FUNCTION "OutputsLoader" : VOID
TITLE =Outputs loader
//Network 1-3 is the startup sequence for the robot cabinet and must not be
//changed in any way
VERSION : 0.1

BEGIN
NETWORK
TITLE =Reset emergency stop loaderside
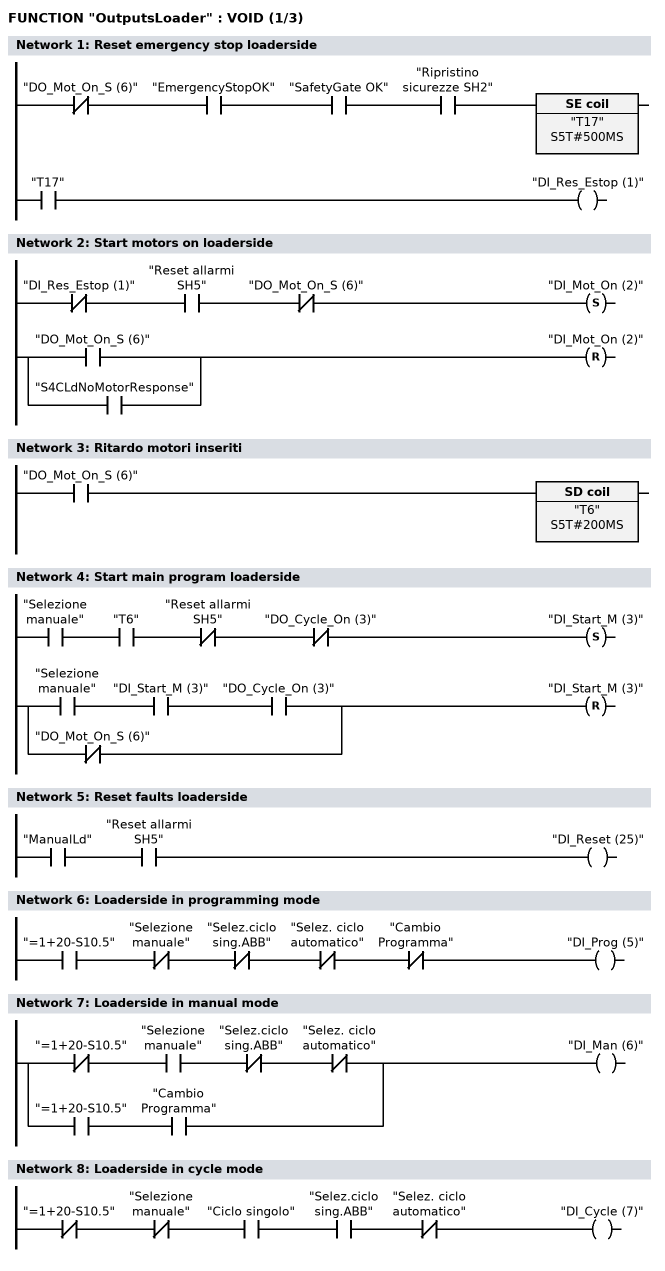
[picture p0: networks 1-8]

      UN    "DO_Mot_On_S (6)";
      U     "EmergencyStopOK";
      U     "SafetyGate OK";
      U     "Ripristino sicurezze SH2";
      L     S5T#500MS;
      SV    "T17";
      NOP   0;
      NOP   0;
      NOP   0;
      U     "T17";
      =     "DI_Res_Estop (1)";
NETWORK
TITLE =Start motors on loaderside

      UN    "DI_Res_Estop (1)";
      U     "Reset allarmi SH5";
      UN    "DO_Mot_On_S (6)";
      S     "DI_Mot_On (2)";
      U(    ;
      O     "DO_Mot_On_S (6)";
      O     "S4CLdNoMotorResponse";
      )     ;
      R     "DI_Mot_On (2)";
      NOP   0;
NETWORK
TITLE =Ritardo motori inseriti

      U     "DO_Mot_On_S (6)";
      L     S5T#200MS;
      SE    "T6";
NETWORK
TITLE =Start main program loaderside

      U     "Selezione manuale";
      U     "T6";
      UN    "Reset allarmi SH5";
      UN    "DO_Cycle_On (3)";
      S     "DI_Start_M (3)";
      U(    ;
      U     "Selezione manuale";
      U     "DI_Start_M (3)";
      U     "DO_Cycle_On (3)";
      ON    "DO_Mot_On_S (6)";
      )     ;
      R     "DI_Start_M (3)";
      NOP   0;
NETWORK
TITLE =Reset faults loaderside

      U     "ManualLd";
      U     "Reset allarmi SH5";
      =     "DI_Reset (25)";
NETWORK
TITLE =Loaderside in programming mode

      U     "=1+20-S10.5";
      UN    "Selezione manuale";
      UN    "Selez.ciclo sing.ABB";
      UN    "Selez. ciclo automatico";
      UN    "Cambio Programma";
      =     "DI_Prog (5)";
NETWORK
TITLE =Loaderside in manual mode

      UN    "=1+20-S10.5";
      U     "Selezione manuale";
      UN    "Selez.ciclo sing.ABB";
      UN    "Selez. ciclo automatico";
      O     ;
      U     "=1+20-S10.5";
      U     "Cambio Programma";
      =     "DI_Man (6)";
NETWORK
TITLE =Loaderside in cycle mode

      UN    "=1+20-S10.5";
      UN    "Selezione manuale";
      U     "Ciclo singolo";
      U     "Selez.ciclo sing.ABB";
      UN    "Selez. ciclo automatico";
      =     "DI_Cycle (7)";
NETWORK
TITLE =Loaderside in auto mode
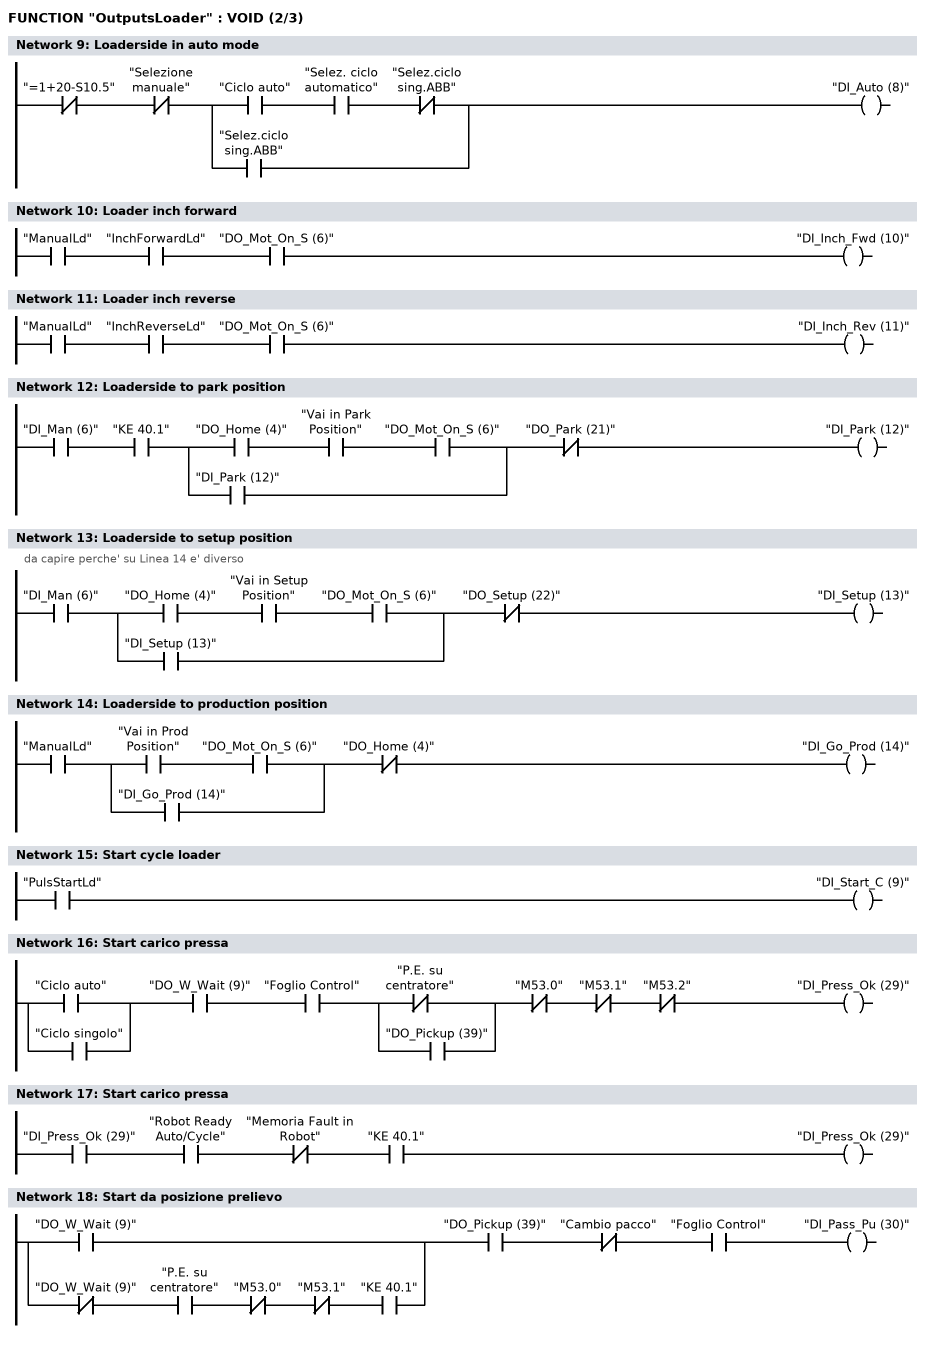
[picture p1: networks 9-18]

      UN    "=1+20-S10.5";
      UN    "Selezione manuale";
      U(    ;
      U     "Ciclo auto";
      U     "Selez. ciclo automatico";
      UN    "Selez.ciclo sing.ABB";
      O     "Selez.ciclo sing.ABB";
      )     ;
      =     "DI_Auto (8)";
NETWORK
TITLE =Loader inch forward

      U     "ManualLd";
      U     "InchForwardLd";
      U     "DO_Mot_On_S (6)";
      =     "DI_Inch_Fwd (10)";
NETWORK
TITLE =Loader inch reverse

      U     "ManualLd";
      U     "InchReverseLd";
      U     "DO_Mot_On_S (6)";
      =     "DI_Inch_Rev (11)";
NETWORK
TITLE =Loaderside to park position

      U     "DI_Man (6)";
      U     "KE 40.1";
      U(    ;
      U     "DO_Home (4)";
      U     "Vai in Park Position";
      U     "DO_Mot_On_S (6)";
      O     "DI_Park (12)";
      )     ;
      UN    "DO_Park (21)";
      =     "DI_Park (12)";
NETWORK
TITLE =Loaderside to setup position
//da capire perche' su Linea 14 e' diverso
      U     "DI_Man (6)";
      U(    ;
      U     "DO_Home (4)";
      U     "Vai in Setup Position";
      U     "DO_Mot_On_S (6)";
      O     "DI_Setup (13)";
      )     ;
      UN    "DO_Setup (22)";
      =     "DI_Setup (13)";
NETWORK
TITLE =Loaderside to production position

      U     "ManualLd";
      U(    ;
      U     "Vai in Prod Position";
      U     "DO_Mot_On_S (6)";
      O     "DI_Go_Prod (14)";
      )     ;
      UN    "DO_Home (4)";
      =     "DI_Go_Prod (14)";
NETWORK
TITLE =Start cycle loader

      U     "PulsStartLd";
      =     "DI_Start_C (9)";
NETWORK
TITLE =Start carico pressa

      U(    ;
      O     "Ciclo auto";
      O     "Ciclo singolo";
      )     ;
      U     "DO_W_Wait (9)";
      U     "Foglio Control";
      U(    ;
      ON    "P.E. su centratore";
      O     "DO_Pickup (39)";
      )     ;
      UN    "M53.0";
      UN    "M53.1";
      UN    "M53.2";
      =     "DI_Press_Ok (29)";
NETWORK
TITLE =Start carico pressa

      U     "DI_Press_Ok (29)";
      U     "Robot Ready Auto/Cycle";
      UN    "Memoria Fault in Robot";
      U     "KE 40.1";
      =     "DI_Press_Ok (29)";
NETWORK
TITLE =Start da posizione prelievo

      U(    ;
      O     "DO_W_Wait (9)";
      O     ;
      UN    "DO_W_Wait (9)";
      U     "P.E. su centratore";
      UN    "M53.0";
      UN    "M53.1";
      U     "KE 40.1";
      )     ;
      U     "DO_Pickup (39)";
      UN    "Cambio pacco";
//      U     "E 10.6"
      U     "Foglio Control";
      =     "DI_Pass_Pu (30)";
NETWORK
TITLE =Foglio singolo Ok al 1° tentativo
//Se non ok entra in rutine di caduta e ripresa materiale.
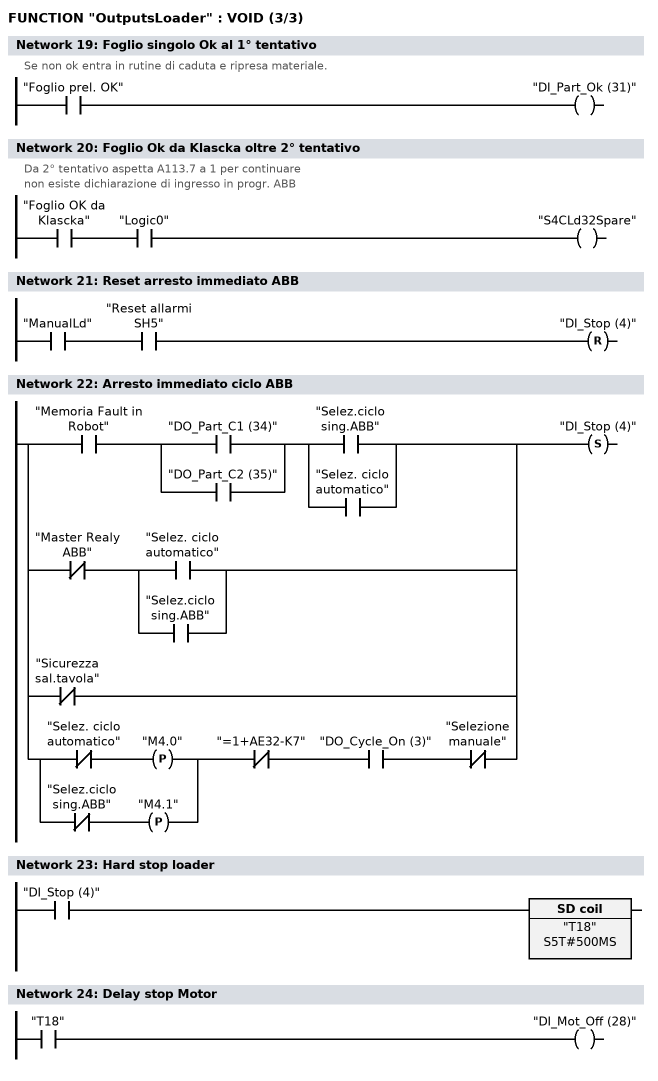
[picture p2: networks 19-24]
      U     "Foglio prel. OK";
      =     "DI_Part_Ok (31)";
NETWORK
TITLE =Foglio Ok da Klascka oltre 2° tentativo
//Da 2° tentativo aspetta A113.7 a 1 per continuare
//non esiste dichiarazione di ingresso in progr. ABB
      U     "Foglio OK da Klascka";
      U     "Logic0";
      =     "S4CLd32Spare";
NETWORK
TITLE =Reset arresto immediato ABB

      U     "ManualLd";
      U     "Reset allarmi SH5";
      R     "DI_Stop (4)";
NETWORK
TITLE =Arresto immediato ciclo ABB

      U     "Memoria Fault in Robot";
      U(    ;
      O     "DO_Part_C1 (34)";
      O     "DO_Part_C2 (35)";
      )     ;
      U(    ;
      O     "Selez.ciclo sing.ABB";
      O     "Selez. ciclo automatico";
      )     ;
      O(    ;
      UN    "Master Realy ABB";
      U(    ;
      O     "Selez. ciclo automatico";
      O     "Selez.ciclo sing.ABB";
      )     ;
      )     ;
      ON    "Sicurezza sal.tavola";
      O(    ;
      U(    ;
      UN    "Selez. ciclo automatico";
      FP    "M4.0";
      O(    ;
      UN    "Selez.ciclo sing.ABB";
      FP    "M4.1";
      )     ;
      )     ;
      UN    "=1+AE32-K7";
      U     "DO_Cycle_On (3)";
      UN    "Selezione manuale";
      )     ;
      S     "DI_Stop (4)";
NETWORK
TITLE =Hard stop loader

      U     "DI_Stop (4)";
      L     S5T#500MS;
      SE    "T18";
      NOP   0;
      NOP   0;
      NOP   0;
      NOP   0;
NETWORK
TITLE =Delay stop Motor

      U     "T18";
      =     "DI_Mot_Off (28)";
END_FUNCTION

